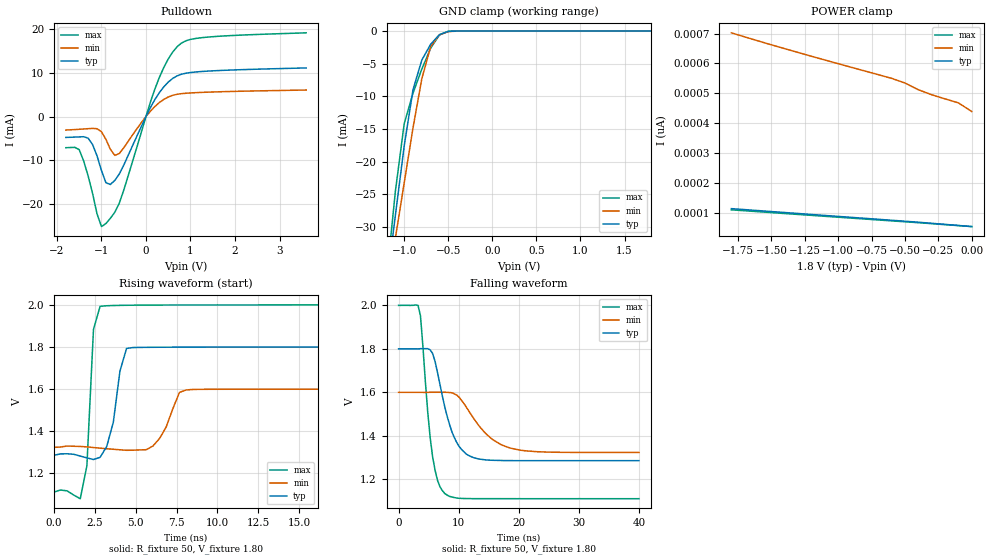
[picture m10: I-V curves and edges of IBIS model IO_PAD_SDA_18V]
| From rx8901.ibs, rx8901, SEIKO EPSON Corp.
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[Model]   IO_PAD_SDA_18V
Model_type I/O_open_drain
Enable Active-High
Polarity Non-Inverting
Vinh=1.26
Vinl=0.54
Vref=2.00
Vmeas=0.90
Rref=5000
C_comp   2.5p   2.0p   3.0p
[Temperature Range] 25   105   -40
[Voltage Range]   1.80   1.60   2.00
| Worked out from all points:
|   slope of the pulldown table from 0 to 0.27 V, typ, clamps not added: 54.4 ohm
|   GND clamp passes 1 mA (typ) near -0.63 V on its own axis
|   falling waveform, R_fixture 50, V_fixture 1.80: 20-80 % time 2.91ns typ, 4.92ns min, 1.74ns max; typ from 1.8 V to 1.29 V
|   rising waveform, R_fixture 50, V_fixture 1.80: 20-80 % time 638ps typ, 910ps min, 332ps max; typ from 1.29 V to 1.8 V
[Pulldown]
-1.8V     -4.763mA   -3.077mA   -7.1mA
-1.5V     -4.644mA   -2.906mA   -7.544mA
-1.2V     -6.372mA   -2.699mA   -17.48mA
-1V       -12.3mA    -3.456mA   -25.07mA
-900mV    -15.07mA   -5.196mA   -24.38mA
-800mV    -15.48mA   -7.459mA   -23.19mA
-600mV    -13.11mA   -8.434mA   -19.76mA
200mV     3.863mA    2.284mA    6.265mA
500mV     7.84mA     4.449mA    13.11mA
700mV     9.268mA    5.071mA    15.9mA
1.3V      10.29mA    5.52mA     18.02mA
3.6V      11.07mA    6.04mA     19.07mA
[GND Clamp]
-1.8V     -104.1mA   -93.3mA    -119.3mA
-1.2V     -38.9mA    -40.17mA   -37.89mA
-1.1V     -28.19mA   -31.69mA   -24.51mA
-1V       -17.59mA   -23.23mA   -14.19mA
-900mV    -8.966mA   -14.81mA   -9.504mA
-800mV    -4.444mA   -7.286mA   -5.814mA
-700mV    -2.032mA   -2.404mA   -2.637mA
-600mV    -545.2uA   -567.3uA   -605.7uA
-500mV    -56.87uA   -91.02uA   -35.51uA
-400mV    -3.146uA   -10.08uA   -733.4nA
1.8V      53.94pA    481.5pA    47.64pA
[POWER Clamp]
-1.8V     114.1pA    702.6pA    110pA
-1.3V     97.76pA    636.7pA    94.59pA
-600mV    75.14pA    550.2pA    73.08pA
-500mV    71.92pA    534.6pA    70.04pA
-400mV    68.56pA    512.2pA    66.99pA
-300mV    64.96pA    495.2pA    63.73pA
-100mV    57.73pA    468.2pA    57.18pA
0V        53.94pA    439.2pA    54.02pA
[Falling Waveform]
R_fixture=50
V_fixture=1.80
V_fixture_min=1.60
V_fixture_max=2.00
0s        1.8V       1.6V       2V
3.232ns   1.8V       1.6V       2V
3.636ns   1.801V     1.6V       1.953V
4.848ns   1.801V     1.6V       1.51V
5.657ns   1.779V     1.6V       1.304V
7.677ns   1.534V     1.6V       1.135V
9.697ns   1.368V     1.587V     1.114V
12.53ns   1.299V     1.479V     1.111V
19.8ns    1.286V     1.337V     1.111V
40ns      1.286V     1.324V     1.111V
[Rising Waveform]
R_fixture=50
V_fixture=1.80
V_fixture_min=1.60
V_fixture_max=2.00
0s        1.286V     1.324V     1.111V
1.616ns   1.282V     1.328V     1.08V
2.02ns    1.274V     1.326V     1.235V
2.424ns   1.266V     1.323V     1.884V
2.828ns   1.276V     1.32V      1.993V
3.636ns   1.443V     1.315V     1.997V
4.444ns   1.793V     1.31V      1.998V
6.061ns   1.799V     1.33V      1.999V
8.081ns   1.8V       1.596V     2V
40ns      1.8V       1.6V       2V
[Ramp]
R_load=50
dV/dt_r   3.085E-1/5.425E-10   1.659E-1/8.792E-10   5.334E-1/3.132E-10
dV/dt_f   3.085E-1/2.900E-9   1.659E-1/4.922E-9   5.334E-1/1.719E-9
|[End   IO_PAD_SDA_18V
